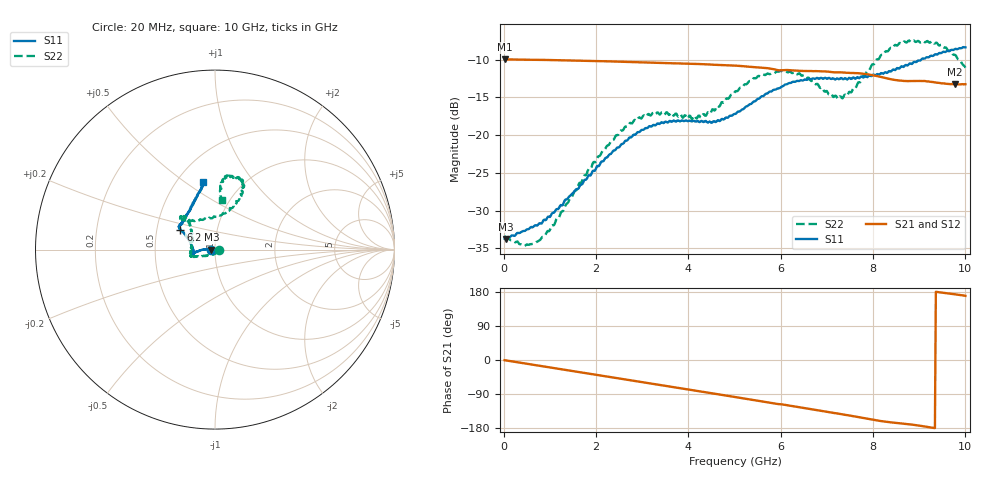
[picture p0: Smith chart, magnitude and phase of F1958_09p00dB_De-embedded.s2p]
! Integrated Device Technology
! Corporate Headquarters
! 6024 Silver Creek Valley Road
! San Jose, CA 95138  USA
! Phone:  1-408-284-8200
! Toll Free:  1-800-223-1366
! Webpage:  http://www.idt.com/
! Timing and RF Division
! 515 Groton Road, Suite 102
! Westford, MA 01886-6024
! Device:  F1958
! Description: 7-bit 0.25 dB Digital Step Attenuator
! Frequency:  0.001 -  6.000 GHz
! Package:  4x4 mm Thin QFN Plastic Package: 24 pin
! Ports:  2 RF, 12 DC
!  Pin  1  = D0
!  Pin  2  = VDD
!  Pin  3  = VMODE
!  Pin  4  = GND
!  Pin  5  = RF1  =  Port 1
!  Pin  6  = GND
!  Pin  7  = GND
!  Pin  8  = GND
!  Pin  9  = GND
!  Pin 10  = GND
!  Pin 11  = GND
!  Pin 12  = GND
!  Pin 13  = GND
!  Pin 14  = RF2  =  Port 2
!  Pin 15  = GND
!  Pin 16  = LE
!  Pin 17  = CLK
!  Pin 18  = DATA
!  Pin 19  = D6
!  Pin 20  = D5
!  Pin 21  = D4
!  Pin 22  = D3
!  Pin 23  = D2
!  Pin 24  = D1
! State:  36
! Atten State:  9.00 dB
! Voltage:  +3.30 Volts
! Current:  0.258 mA
! Data:  The device was measured on a F1958 evaluation board which has
!  individual transmission lines to the RF pins.  Data was collected
!  using a calibrated network analyzer.  The evaluation board was
!  de-embedded using Automatic Fixture Removal (AFR).
!  The reference plane is the edge of the package pin.
! Misc:
!  Action Tracker AT0419
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# GHz S dB R 50
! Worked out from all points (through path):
!   500 points, 20 MHz to 10 GHz, reference 50 ohm
!   highest |S21| = -9.93 dB at 20 MHz (marker M1); lowest = -13.3 dB at 9.78 GHz (marker M2)
!   group delay of S21, straight-line fit = 53.7 ps
!   lowest |S11| = -33.8 dB at 40 MHz (marker M3), VSWR 1.04, Z = 48 - j0.0762 ohm
!   |S11| at or under -10 dB: start of sweep to 9.042 GHz
!   |S22| runs from -34.7 to -7.4 dB; largest |S21 - S12| = 0.00092
!   S11 on the Smith chart (normalised r, x): 20 MHz: 0.96, -0.00; 6.2 GHz: 0.66, +0.15; 10 GHz: 0.67, +0.59
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0.02  -33.71 -177.9  -9.93 -0.5  -9.93 -0.5  -33.34 -5.8
0.04  -33.76 -177.8  -9.94 -0.9  -9.94 -0.9  -33.54 -8.9
0.44  -32.69 174.6  -9.99 -8.7  -9.99 -8.7  -34.72 -37.6
0.76  -31.74 174.1  -10.01 -14.9  -10.01 -14.9  -34.00 -67.7
1.1  -30.21 175.7  -10.04 -21.6  -10.04 -21.5  -31.83 -101.0
1.7  -26.51 178.5  -10.12 -33.2  -10.11 -33.1  -26.02 -139.5
2.58  -21.15 -175.1  -10.27 -50.3  -10.26 -50.3  -19.37 -159.2
2.92  -19.59 -172.7  -10.33 -56.9  -10.32 -57.0  -17.70 -162.6
3.36  -18.50 -170.1  -10.43 -65.4  -10.43 -65.5  -17.15 -165.2
4.24  -18.27 -174.0  -10.57 -82.5  -10.58 -82.6  -17.41 166.3
5.02  -17.18 166.2  -10.78 -97.9  -10.79 -97.9  -14.17 135.9
5.54  -15.12 155.1  -11.02 -108.2  -11.03 -108.2  -12.17 133.2
6.2  -13.07 150.3  -11.39 -120.6  -11.40 -120.6  -11.57 137.4
6.68  -12.51 147.5  -11.50 -129.8  -11.52 -129.8  -12.78 133.6
7.1  -12.55 143.6  -11.63 -138.9  -11.64 -138.7  -14.54 115.8
7.36  -12.58 141.2  -11.69 -144.0  -11.70 -143.9  -14.91 92.7
7.9  -12.18 130.9  -11.94 -155.6  -11.94 -155.6  -11.34 67.8
8.34  -11.53 121.4  -12.52 -163.9  -12.53 -164.0  -8.74 64.4
8.74  -10.76 113.9  -12.83 -169.0  -12.83 -169.0  -7.66 69.0
9.24  -9.50 104.8  -12.92 -178.1  -12.93 -178.1  -7.70 79.3
9.78  -8.56 100.4  -13.27 173.2  -13.29 173.2  -9.36 84.4
10  -8.36 100.1  -13.24 169.2  -13.27 169.4  -11.06 82.1
